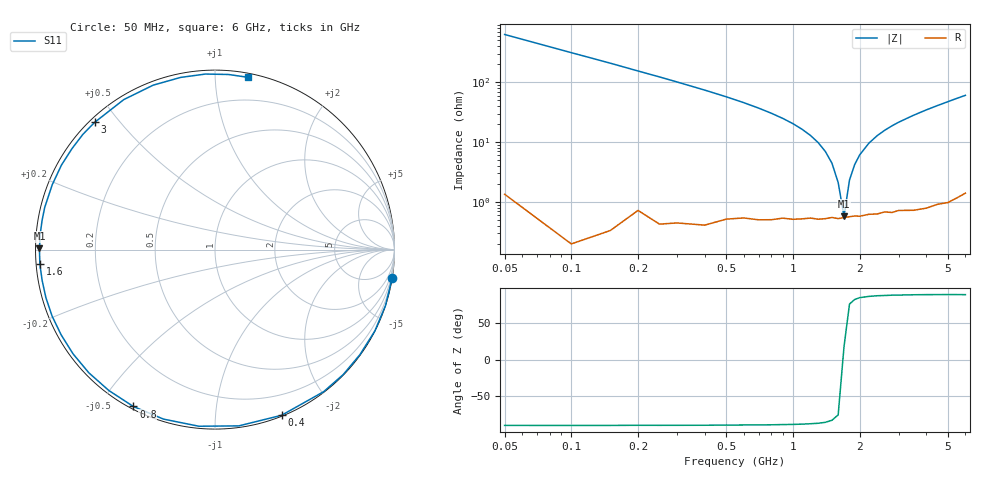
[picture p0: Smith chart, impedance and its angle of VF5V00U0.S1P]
! Infineon Technologies  Discrete & RF Semiconductors
! BBY 58-03
! Si Tuning Diode in SOD323
! VR = 5 V
! S-Parameters:  June  1999
# GHz  S  MA  R  50
!  f  S11
! GHz  MAG  ANG
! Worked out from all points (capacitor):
!   34 points, 50 MHz to 6 GHz, reference 50 ohm
!   read as one part to ground: C = 5.06 pF near 50 MHz
!   lowest |Z| = 578 mohm at 1.7 GHz (marker M1)
!   series resonance near 1.692 GHz, so ESL is about 1.7 nH
!   S11 on the Smith chart (normalised r, x): 50 MHz: 0, -13; 400 MHz: 0.01, -1.48; 800 MHz: 0.01, -0.61; 1.6 GHz: 0.01, -0.04; 3 GHz: 0.01, +0.43; 6 GHz: 0.03, +1.21
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0.05  0.9997 -9.1
0.1  0.9998 -18.2
0.15  0.9993 -27.0
0.2  0.9972 -35.9
0.25  0.9976 -44.3
0.3  0.9965 -52.6
0.4  0.9949 -68.1
0.5  0.9911 -82.3
0.6  0.9882 -95.2
0.7  0.987 -106.9
0.8  0.9853 -117.5
0.9  0.9829 -127.0
1  0.9825 -135.7
1.1  0.9812 -143.7
1.2  0.9799 -151.0
1.4  0.9795 -164.1
1.6  0.9791 -175.3
1.7  0.9782 179.6
2  0.9774 166.1
2.4  0.9765 151.2
2.8  0.9768 138.9
3  0.9759 133.4
3.5  0.9781 121.3
4  0.9788 110.6
4.5  0.9782 101.3
5  0.9795 93.1
5.5  0.9785 85.6
6  0.9774 79.1
